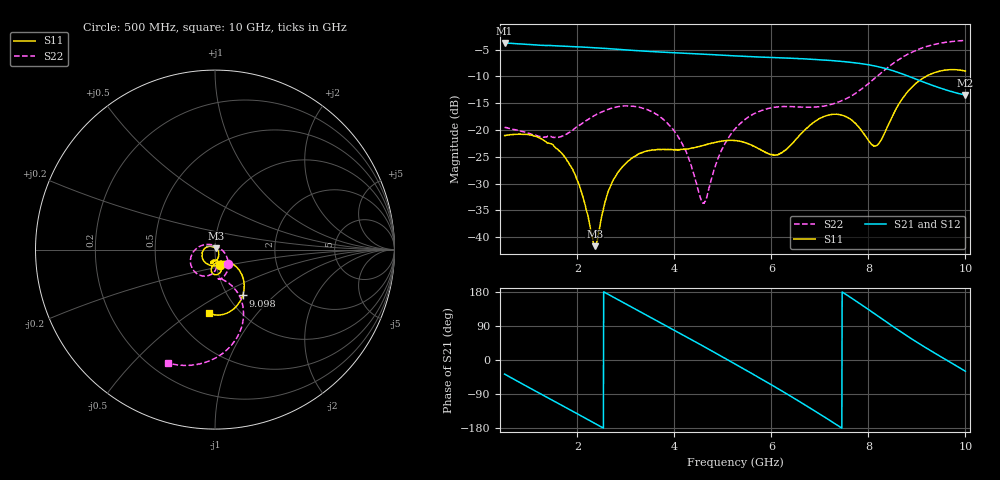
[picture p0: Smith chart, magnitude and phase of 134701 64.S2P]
!  2-Port S-parameters saved by WinCal
! VAR MeasName=S-Parameters (CALIBRATED_DATA) read from VNA (N5242A)
! VAR MeasDate=2013-7-3 16:41:52
! VAR NAME=134701 64
! VAR FILENAME=134701 64.S2P
! VAR DATE=2013-7-3 16:41:52
! VAR PHYS_PORTS=1,2
# Hz S MA R 50
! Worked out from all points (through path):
!   1601 points, 500 MHz to 10 GHz, reference 50 ohm
!   highest |S21| = -3.76 dB at 500 MHz (marker M1); lowest = -13.5 dB at 9.994 GHz (marker M2)
!   group delay of S21, straight-line fit = 208 ps
!   lowest |S11| = -41.7 dB at 2.358 GHz (marker M3), VSWR 1.02, Z = 50.5 + j0.67 ohm
!   |S11| at or under -10 dB: start of sweep to 9.189 GHz
!   |S22| runs from -33.7 to -3.3 dB; largest |S21 - S12| = 0.0016
!   S11 on the Smith chart (normalised r, x): 500 MHz: 1.04, -0.18; 9.098 GHz: 1.17, -0.65; 10 GHz: 0.73, -0.59
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5e8  0.08883 -73.5  0.6488 -37.2  0.6481 -37.2  0.1059 -47.0
9.096875e8  0.09118 -117.6  0.6305 -66.2  0.6307 -66.2  0.09567 -72.9
1.277812e9  0.08172 -151.3  0.6153 -91.7  0.6154 -91.7  0.08623 -84.5
1.729062e9  0.05704 172.2  0.6023 -123.1  0.6025 -123.1  0.08933 -85.6
2.085312e9  0.02642 137.9  0.5934 -148.0  0.5933 -148.0  0.114 -88.6
2.358438e9  0.008264 53.4  0.5834 -167.2  0.5836 -167.3  0.1369 -97.1
2.61375e9  0.02497 -34.7  0.5743 174.9  0.5746 174.9  0.1546 -107.9
2.8275e9  0.03969 -57.8  0.5657 159.9  0.5654 159.9  0.1645 -118.6
3.249062e9  0.05926 -81.3  0.5482 130.7  0.5484 130.6  0.1643 -141.0
3.670625e9  0.06586 -95.9  0.5349 101.5  0.5335 101.5  0.1361 -165.2
4.169375e9  0.0661 -99.9  0.5202 66.6  0.5196 66.6  0.07328 160.9
4.596875e9  0.07188 -98.5  0.5084 36.4  0.5089 36.4  0.02078 65.4
4.94125e9  0.07846 -100.9  0.4997 11.7  0.4998 11.8  0.06043 -21.5
5.25e9  0.07985 -105.4  0.4908 -10.5  0.4914 -10.6  0.1024 -43.9
6.093125e9  0.0585 -90.2  0.4724 -72.4  0.4726 -72.5  0.1635 -77.0
6.835312e9  0.1142 -71.6  0.4564 -129.8  0.4567 -129.7  0.163 -82.0
7.5775e9  0.1304 -97.2  0.43 169.7  0.4307 169.6  0.1994 -68.2
8.12375e9  0.07082 -76.0  0.3959 122.3  0.3964 122.3  0.3015 -62.3
8.420625e9  0.1141 -40.8  0.3669 96.2  0.3665 96.1  0.3881 -65.8
9.0975e9  0.2984 -58.8  0.2848 39.2  0.2843 39.1  0.5798 -85.8
9.994062e9  0.355 -95.0  0.2117 -29.2  0.2119 -29.4  0.6832 -112.2
1e10  0.3548 -95.2  0.2119 -29.7  0.2117 -29.9  0.6834 -112.3
